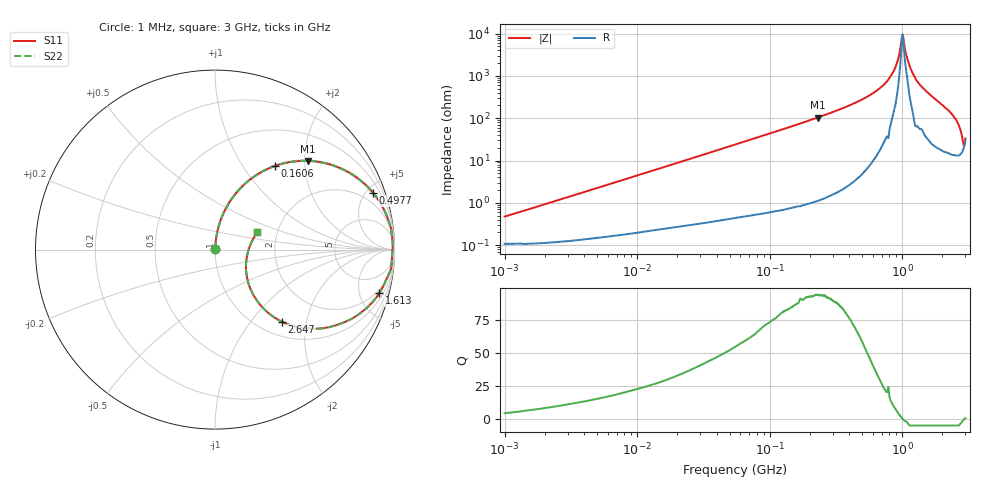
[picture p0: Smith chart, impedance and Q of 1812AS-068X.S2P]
!s-Parameter Generated by FASTRON Sdn. Bhd.
!FASTRON P/N : 1812AS-068X
!Keysight Technologies,E4991B,MY54100416,A.01.15
!Date created: Fri Oct 13 14:23:45 2023
!Version  : Rev00 Fri Oct 13 14:23:45 2023
!Data & Calibration Information:
!Freq	S11	S21	S12	S22
!PortZ  Port1:50+j0  Port2:50+j0
!When reading, reference impedance value at option line is always used.
! Remarks : This data is being provided solely for informational purposes.
# Hz S dB R 50
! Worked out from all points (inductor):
!   1601 points, 1 MHz to 3 GHz, reference 50 ohm
!   read as one part in series: L = 73 nH near 1.041 MHz
!   highest Q = 93.6 at 230.3 MHz (marker M1), where L = 71.7 nH
!   self-resonance near 1.008 GHz
!   S11 on the Smith chart (normalised r, x): 1 MHz: 1.00, +0.01; 160.6 MHz: 1.02, +1.41; 497.7 MHz: 1.09, +5.54; 1.613 GHz: 1.56, -7.31; 2.647 GHz: 1.26, -1.45; 3 GHz: 1.57, +0.33
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1000000  -46.54 76.6  -0.01 -0.3  -0.01 -0.3  -46.54 76.6
3804036  -35.31 84.5  -0.01 -1.0  -0.01 -1.0  -35.31 84.5
1.447069e7  -23.97 84.3  -0.04 -3.6  -0.04 -3.6  -23.97 84.3
5.477226e7  -12.76 75.6  -0.27 -13.3  -0.27 -13.3  -12.76 75.6
1.606197e8  -4.82 54.3  -1.80 -35.0  -1.80 -35.0  -4.82 54.3
2.083556e8  -3.38 46.7  -2.76 -42.7  -2.76 -42.7  -3.38 46.7
2.302869e8  -2.90 43.6  -3.22 -45.8  -3.22 -45.8  -2.90 43.6
4.976708e8  -0.58 19.7  -9.43 -69.3  -9.43 -69.3  -0.58 19.7
6.553423e8  -0.25 11.9  -13.70 -76.3  -13.70 -76.3  -0.25 11.9
7.925923e8  -0.11 6.7  -18.70 -80.7  -18.70 -80.7  -0.11 6.7
8.982141e8  -0.09 3.2  -24.87 -78.5  -24.87 -78.5  -0.09 3.2
9.828732e8  -0.09 0.7  -35.96 -51.9  -35.96 -51.9  -0.09 0.7
1.007775e9  -0.09 0.0  -39.70 -1.7  -39.70 -1.7  -0.09 0.0
1.033307e9  -0.10 -0.7  -35.57 45.9  -35.57 45.9  -0.10 -0.7
1.11944e9  -0.11 -2.7  -26.20 73.7  -26.20 73.7  -0.11 -2.7
1.22495e9  -0.12 -5.5  -20.38 79.1  -20.38 79.1  -0.12 -5.5
1.347129e9  -0.22 -8.7  -16.36 76.2  -16.36 76.2  -0.22 -8.7
1.613037e9  -0.48 -14.9  -11.76 70.7  -11.76 70.7  -0.48 -14.9
2.167021e9  -1.68 -29.5  -6.11 55.1  -6.11 55.1  -1.68 -29.5
2.647227e9  -5.21 -47.1  -2.57 32.7  -2.57 32.7  -5.21 -47.1
2.86789e9  -12.10 -43.1  -1.55 11.7  -1.55 11.7  -12.10 -43.1
3e9  -11.89 22.3  -2.26 -7.2  -2.26 -7.2  -11.89 22.3
